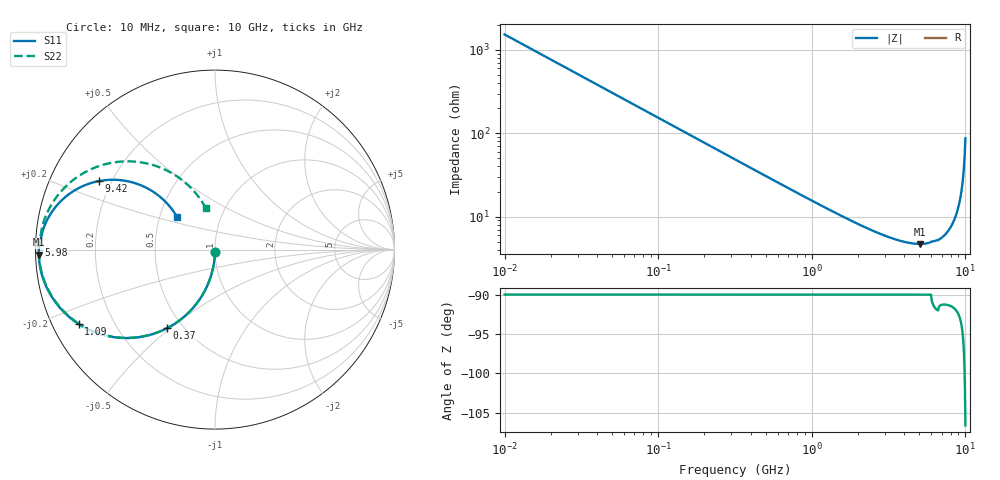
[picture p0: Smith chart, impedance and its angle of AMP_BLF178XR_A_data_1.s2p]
! Created Wed Jun 13 16:06:13 2012
# ghz S ma R 50
! 2 Port Network Data from SP1.SP block
! freq  magS11  angS11  magS21  angS21  magS12  angS12  magS22  angS22
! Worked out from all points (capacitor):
!   1000 points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, 10 MHz to 10 GHz, reference 50 ohm
!   read as one part in shunt: C = 10.4 pF near 60 MHz
!   lowest |Z| = 4.71 ohm at 5.06 GHz (marker M1)
!   S11 on the Smith chart (normalised r, x): 10 MHz: 1.00, -0.03; 370 MHz: 0.41, -0.49; 1.09 GHz: 0.08, -0.25; 5.98 GHz: 0.01, +0.01; 9.42 GHz: 0.15, +0.27; 10 GHz: 0.62, +0.24
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0.01  0.01615 -90.9  0.9999 -0.9  0.9999 -0.9  0.01615 -90.9
0.08  0.1282 -97.5  0.9917 -7.5  0.9917 -7.5  0.1282 -97.5
0.13  0.2055 -102.0  0.9787 -12.0  0.9787 -12.0  0.2055 -102.1
0.23  0.3481 -110.7  0.9375 -20.7  0.9375 -20.7  0.3481 -110.7
0.37  0.5123 -121.3  0.8588 -31.4  0.8588 -31.4  0.5123 -121.4
0.52  0.6417 -130.6  0.767 -40.7  0.767 -40.7  0.6417 -130.7
0.72  0.7557 -140.0  0.6549 -50.1  0.6549 -50.1  0.7557 -140.2
1.09  0.8657 -151.4  0.5006 -61.6  0.5006 -61.6  0.8657 -151.7
1.68  0.9333 -161.3  0.3591 -71.5  0.3591 -71.5  0.9333 -161.7
2.45  0.9636 -168.0  0.2674 -78.3  0.2674 -78.3  0.9636 -168.7
3.34  0.9763 -172.6  0.2163 -83.1  0.2163 -83.1  0.9763 -173.5
5.01  0.9824 -178.2  0.1867 -89.0  0.1867 -89.0  0.9824 -179.8
5.06  0.9824 -178.4  0.1867 -89.2  0.1867 -89.2  0.9824 180.0
5.98  0.9802 178.5  0.1976 -92.5  0.1976 -92.5  0.9802 176.5
6.67  0.9709 176.7  0.2059 -96.4  0.2059 -96.4  0.9731 174.2
8.34  0.9353 167.4  0.3259 -106.6  0.3259 -106.6  0.9365 162.8
8.97  0.8737 159.6  0.4499 -116.1  0.4499 -116.1  0.8743 153.1
9.42  0.7522 149.5  0.6113 -129.2  0.6113 -129.2  0.7504 139.8
9.61  0.651 143.6  0.7051 -137.9  0.7051 -137.9  0.6462 131.0
9.76  0.5348 138.6  0.7857 -146.7  0.7857 -146.7  0.5249 121.9
9.87  0.4254 136.1  0.8422 -154.4  0.8422 -154.4  0.4082 113.9
10  0.2767 139.5  0.8952 -164.9  0.8952 -164.9  0.239 102.7
